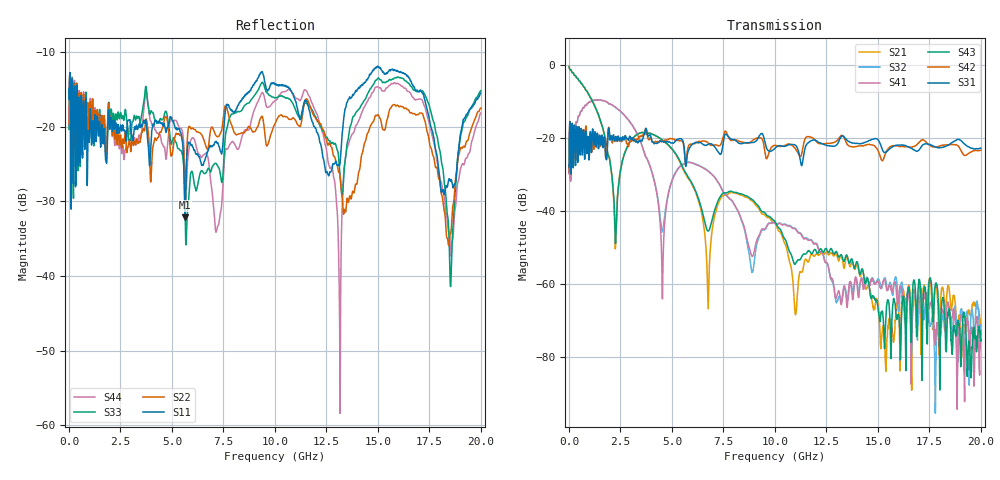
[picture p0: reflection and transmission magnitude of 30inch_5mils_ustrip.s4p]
! FILE: C:\Archive\FR4 ustrip trace\5mils\30inch_5mils_ustrip.s4p
# MHz S DB R 50.00
! FREQ  S11  S12  S13  S14
!  S21  S22  S23  S24
!  S31  S32  S33  S34
!  S41  S42  S43  S44
!  DB  ANG  DB  ANG  DB  ANG  DB  ANG
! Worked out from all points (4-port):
!   2000 points, 10 MHz to 20 GHz, reference 50 ohm
!   strongest paths, dB at 10 MHz, 5.01 GHz, 10.01 GHz, 15.01 GHz, 20 GHz:
!     S31: -27.9, -21.3, -22.7, -20.4, -22.7
!     S42: -29.1, -20.1, -22.0, -23.4, -23.3
!     S43: -0.4, -22.9, -42.9, -66.7, -75.4
!     S41: -29.4, -31.6, -43.4, -59.3, -72.7
!     S32: -27.1, -31.4, -43.2, -58.6, -71.1
!     S21: -0.2, -23.1, -43.2, -65.5, -71.1
!   lowest |S11| = -32.1 dB at 5.64 GHz (marker M1), VSWR 1.05, Z = 49.2 - j2.32 ohm
!   |S11| at or under -10 dB: start of sweep to end of sweep
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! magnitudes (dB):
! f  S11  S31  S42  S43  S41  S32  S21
! 10 MHz  -15.0  -27.9  -29.1  -0.4  -29.4  -27.1  -0.2
! 2.25 GHz  -19.7  -20.1  -20.2  -48.2  -11.5  -11.5  -50.3
! 4.54 GHz  -19.5  -20.8  -20.7  -20.4  -64.1  -45.7  -20.5
! 5.64 GHz  -32.1  -25.9  -26.1  -29.2  -27.0  -26.8  -29.6
! 6.76 GHz  -23.2  -21.7  -21.3  -45.4  -29.0  -28.9  -66.8
! 7.95 GHz  -18.0  -20.3  -20.5  -34.7  -37.4  -37.4  -34.9
! 20 GHz  -15.5  -22.7  -23.3  -75.4  -72.7  -71.1  -71.1
